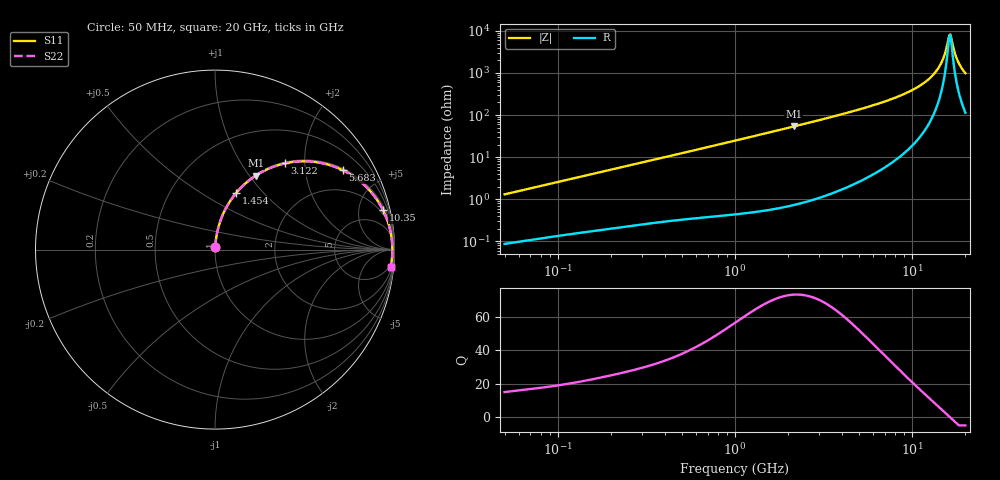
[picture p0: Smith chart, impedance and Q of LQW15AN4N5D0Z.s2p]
!Murata Part Number: LQW15AN4N5D0Z
!These Parameters are Measured in Series Mode Connection
!  o--[Z]--o
!Port1  Port2
!  o-------o
!Freq. Start=50[MHz] Stop=20[GHz], 401[Steps]
# Hz S RI R 50
!Freq.(Hz) S11(Real) S11(Imag) S21(Real) S21(Imag) S12(Real) S12(Imag) S22(Real) S22(Imag)
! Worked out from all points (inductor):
!   401 points, 50 MHz to 20 GHz, reference 50 ohm
!   read as one part in series: L = 4.14 nH near 51.52 MHz
!   highest Q = 73.5 at 2.147 GHz (marker M1), where L = 3.98 nH
!   self-resonance near 16.22 GHz
!   S11 on the Smith chart (normalised r, x): 50 MHz: 1.00, +0.03; 1.454 GHz: 1.01, +0.72; 3.122 GHz: 1.02, +1.59; 5.683 GHz: 1.07, +3.17; 10.35 GHz: 1.43, +8.44; 20 GHz: 3, -20
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5e7  0.00104 0.0131  0.999 -0.0131  0.999 -0.0131  0.00104 0.0131
1.364002e8  0.00281 0.0346  0.9972 -0.0346  0.9972 -0.0346  0.00281 0.0346
3.721004e8  0.0113 0.0915  0.9887 -0.0915  0.9887 -0.0915  0.0113 0.0915
1e9  0.0613 0.2311  0.9387 -0.2311  0.9387 -0.2311  0.0613 0.2311
1.454215e9  0.1187 0.3161  0.8813 -0.3161  0.8813 -0.3161  0.1187 0.3161
2.146657e9  0.2268 0.412  0.7732 -0.412  0.7732 -0.412  0.2268 0.412
2.728004e9  0.3244 0.4613  0.6756 -0.4613  0.6756 -0.4613  0.3244 0.4613
3.121702e9  0.3893 0.4804  0.6107 -0.4804  0.6107 -0.4804  0.3893 0.4804
4.212059e9  0.5502 0.4891  0.4498 -0.4891  0.4498 -0.4891  0.5502 0.4891
5.683258e9  0.7117 0.4424  0.2883 -0.4424  0.2883 -0.4424  0.7117 0.4424
7.442007e9  0.8343 0.3575  0.1657 -0.3575  0.1657 -0.3575  0.8343 0.3575
1.034674e10  0.937 0.2187  0.063 -0.2187  0.063 -0.2187  0.937 0.2187
1.220001e10  0.9674 0.1417  0.0326 -0.1417  0.0326 -0.1417  0.9674 0.1417
1.375312e10  0.981 0.0843  0.019 -0.0843  0.019 -0.0843  0.981 0.0843
1.482269e10  0.986 0.0481  0.014 -0.0481  0.014 -0.0481  0.986 0.0481
1.527346e10  0.9872 0.0335  0.0128 -0.0335  0.0128 -0.0335  0.9872 0.0335
1.597544e10  0.9882 0.0117  0.0118 -0.0117  0.0118 -0.0117  0.9882 0.0117
1.621653e10  0.9883 0.00441  0.0117 -0.00441  0.0117 -0.00441  0.9883 0.00441
1.670968e10  0.9883 -0.0102  0.0117 0.0102  0.0117 0.0102  0.9883 -0.0102
1.747767e10  0.9874 -0.032  0.0126 0.032  0.0126 0.032  0.9874 -0.032
1.828096e10  0.9855 -0.0538  0.0145 0.0538  0.0145 0.0538  0.9855 -0.0538
2e10  0.9788 -0.0972  0.0212 0.0972  0.0212 0.0972  0.9788 -0.0972
